(* Process data send to or received from IEC 60870-5-101 master device (LowLevelMasterSample101 project) *)
TYPE ST_IEC870_5_101SProcData :
STRUCT
	(* Monitoring data points send to IEC 60870-5-101 master device *)
	stSiq100		: ST_IEC870_5_101SIQ;(* Single point information + quality flags, M_SP_NA_1, IOA = 100 *)
	stSiq101		: ST_IEC870_5_101SIQ;(* Single point information + quality flags, M_SP_TA_1, IOA = 101 *)
	stSiq102		: ST_IEC870_5_101SIQ;(* Single point information + quality flags, M_SP_TB_1, IOA = 102 *)
	
	stDiq200		: ST_IEC870_5_101DIQ;(* Double point information + quality flags, M_DP_NA_1, IOA = 200 *)
	
	nVti300			: BYTE := 0;(* Regulating step value, M_ST_NA_1, IOA = 300 *)
	stQds300		: ST_IEC870_5_101QDS;(* Regulating step quality descriptor *)
	
	nBsi400			: DWORD := 0;(* Bitstring value, M_BO_NA_1, IOA = 400 *)
	stQds400		: ST_IEC870_5_101QDS;(* Bitstring quality descriptor *)
	
	nNva500			: WORD := 0;(* Measured value, normalized value, M_ME_NA_1, IOA = 500 *)
	stQds500		: ST_IEC870_5_101QDS;(* Measured value quality descriptor *)

	nSva600			: INT := 0;(* Mesured value, scaled value, M_ME_NB_1, IOA = 600 *)
	stQds600		: ST_IEC870_5_101QDS;(* Measured value quality descriptor *)

	fSingle700		: REAL := 0.0;(* Measured value, short floating point value, M_ME_NC_1, IOA = 700 *)
	stQds700		: ST_IEC870_5_101QDS;(* Measured value quality descriptor *)
	
	nBcr800			: DINT := 0;(* Binary counter value, M_IT_NA_1, IOA = 800 *)
	stQcr800		: ST_IEC870_5_101QCR;(* Binary counter quality descriptor *)

	nBcr801			: DINT := 0;(* Binary counter value, M_IT_TA_1, IOA = 801 *)
	stQcr801		: ST_IEC870_5_101QCR;(* Binary counter quality descriptor *)

	nBcr802			: DINT := 0;(* Binary counter value, M_IT_TB_1, IOA = 802 *)
	stQcr802		: ST_IEC870_5_101QCR;(* Binary counter quality descriptor *)

	(*  Commands received from IEC 60870-5-101 master device *)
	eScs10			: E_IEC870_5_101SCS := eIEC870_SCS_OFF;(* Single command state, C_SC_NA_1, IOA = 10 *)
	eQu10		 	: E_IEC870_5_101QU := eIEC870_QU_UNSPECIFIED;(* Single command qualifier *)
	eCtrl10 		: E_IEC870_5_101CommandState := eIEC870_CMD_NONE;(* Command exeuction/activation control variable *)
	
	eDcs20			: E_IEC870_5_101DCS := eIEC870_DCS_OFF;(* Double command state, C_DC_NA_1, IOA = 20 *)
	eQu20			: E_IEC870_5_101QU := eIEC870_QU_UNSPECIFIED;(* Double command qualifier *)
	eCtrl20 		: E_IEC870_5_101CommandState := eIEC870_CMD_NONE;(* Command exeuction/activation control variable *)

	nVti30			: BYTE := 0;(* Regulating step value, C_RC_NA_1, IOA = 30 *)
	eRcs30			: E_IEC870_5_101RCS := eIEC870_RCS_NOTALLOWED0;(* Regulating step command state *)
	eQu30			: E_IEC870_5_101QU := eIEC870_QU_UNSPECIFIED;(* Regulating step command qualifier *)
	eCtrl30 		: E_IEC870_5_101CommandState := eIEC870_CMD_NONE;(* Command exeuction/activation control variable *)

	nBsi40			: DWORD := 0;(* Binary state information, C_BO_NA_1, IOA = 40 *)
	eCtrl40 		: E_IEC870_5_101CommandState := eIEC870_CMD_NONE;(* Command exeuction/activation control variable *)
	
	nNva50			: WORD := 0;(* Setpoint value, normlized value, C_SE_NA_1, IOA = 50 *)
	eQl50			: E_IEC870_5_101QL := eIEC870_QL_DEFAULT;(* Qualifier of setpoint command *)
	eCtrl50 		: E_IEC870_5_101CommandState := eIEC870_CMD_NONE;(* Command exeuction/activation control variable *)

	nSva60			: INT := 0;(* Setpoint value, scalled value, C_SE_NB_1, IOA = 60 *)
	eQl60			: E_IEC870_5_101QL := eIEC870_QL_DEFAULT;(* Qualifier of setpoint command *)
	eCtrl60 		: E_IEC870_5_101CommandState := eIEC870_CMD_NONE;(* Command exeuction/activation control variable *)

	fSingle70		: REAL := 0;(* Setpoint value, short floating point value, C_SE_NC_1, IOA = 70 *)
	eQl70			: E_IEC870_5_101QL := eIEC870_QL_DEFAULT;(* Qualifier of setpoint command *)
	eCtrl70 		: E_IEC870_5_101CommandState := eIEC870_CMD_NONE;(* Command exeuction/activation control variable *)
	
END_STRUCT
END_TYPE
